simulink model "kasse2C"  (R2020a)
settings: Solver=ode45  StartTime=0.0  StopTime=100  FixedStep=0.001  MaxStep=2  RelTol=1e-3  EnableMultiTasking=on
libraries: simulink x2

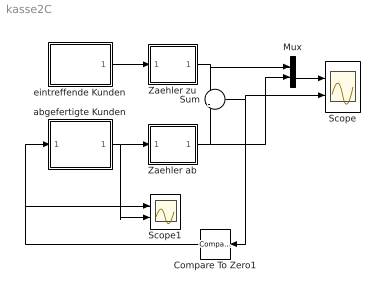
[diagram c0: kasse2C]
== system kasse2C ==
  Compare To Zero1 : simulink/Logic and Bit Operations/Compare To Zero  relop=<=  OutDataTypeStr=uint8
  Mux : Mux  Inputs=2
  Scope : Scope  NumInputPorts=2
  Scope1 : Scope  NumInputPorts=2
  Sum : Sum  Inputs=+|-
  Zaehler ab : Subsystem  mask(Vorwaertszaehler){z0=0}
      mask prompts: z0 "Anfangswert"
      mask help: Einfacher Vorwaertszaehler, getriggert durch Signalabfall
  Zaehler zu : Subsystem  mask(Vorwaertszaehler){z0=0}
      mask prompts: z0 "Anfangswert"
      mask help: Einfacher Vorwaertszaehler, getriggert durch Signalabfall
  abgefertigte Kunden : Subsystem  mask{tAb=1}
      mask prompts: tAb "Abfertigungszeit [s]"
  eintreffende Kunden : Subsystem  mask(Poisson-Impulse){lambda=0.8}
      mask help: Erzeugt Impulse, deren zeitlicher Abstand exponentialverteilt ist mit Rate lambda. Summiert man die Anzahl der Impulse, erhaelt man einen Poisson-Prozess.
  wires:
  Zaehler zu/1(Out) -> Sum/1, Mux/1
  eintreffende Kunden/1(Out1) -> Zaehler zu/1(In)
  abgefertigte Kunden/1(Out) -> Scope1/2, Zaehler ab/1(In)
  Zaehler ab/1(Out) -> Sum/2, Mux/2
  Sum/1 -> Compare To Zero1/1, Scope/2
  Compare To Zero1/1 -> abgefertigte Kunden/1(In1), Scope1/1
  Mux/1 -> Scope/1

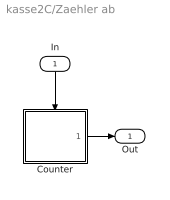
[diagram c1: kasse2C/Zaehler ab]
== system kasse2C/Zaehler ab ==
  In : Inport
  Counter : Subsystem
  Out : Outport
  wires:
  Counter/1(Out) -> Out/1
  In/1 -> Counter/Trigger

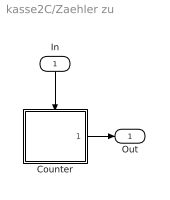
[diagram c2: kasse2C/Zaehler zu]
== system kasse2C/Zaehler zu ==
  In : Inport
  Counter : Subsystem
  Out : Outport
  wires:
  In/1 -> Counter/Trigger
  Counter/1(Out) -> Out/1

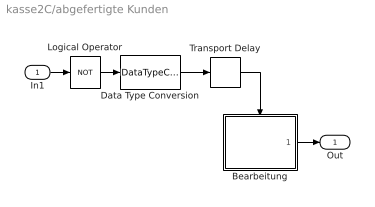
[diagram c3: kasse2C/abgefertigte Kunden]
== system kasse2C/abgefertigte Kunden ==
  In1 : Inport
  Bearbeitung : Subsystem
  Data Type Conversion : DataTypeConversion  OutDataTypeStr=double
  Logical Operator : Logic  Operator=NOT  AllPortsSameDT=off  OutDataTypeStr=boolean
  Transport Delay : TransportDelay  DelayTime=0.2*tAb
  Out : Outport
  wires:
  In1/1 -> Logical Operator/1
  Bearbeitung/1(Out1) -> Out/1
  Logical Operator/1 -> Data Type Conversion/1
  Data Type Conversion/1 -> Transport Delay/1
  Transport Delay/1 -> Bearbeitung/Enable

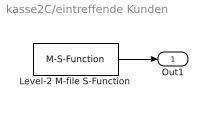
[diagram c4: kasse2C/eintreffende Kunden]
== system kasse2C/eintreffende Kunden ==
  Level-2 M-file S-Function : M-S-Function  FunctionName=sfun_poisson  Parameters=lambda
  Out1 : Outport
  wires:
  Level-2 M-file S-Function/1 -> Out1/1

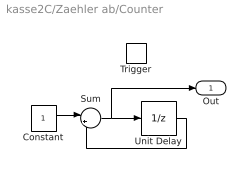
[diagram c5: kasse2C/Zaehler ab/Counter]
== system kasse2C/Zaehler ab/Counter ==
  Trigger : TriggerPort  TriggerType=falling  VariantControl=Variant
  Constant : Constant
  Sum : Sum  Inputs=|++
  Unit Delay : UnitDelay  InitialCondition=z0  SampleTime=-1  HasFrameUpgradeWarning=on
  Out : Outport  InitialOutput=z0
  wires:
  Constant/1 -> Sum/1
  Sum/1 -> Unit Delay/1, Out/1
  Unit Delay/1 -> Sum/2

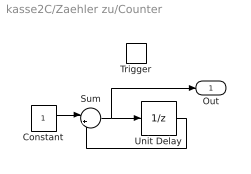
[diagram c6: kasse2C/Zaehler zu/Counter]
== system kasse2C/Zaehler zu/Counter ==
  Trigger : TriggerPort  TriggerType=falling  VariantControl=Variant
  Constant : Constant
  Sum : Sum  Inputs=|++
  Unit Delay : UnitDelay  InitialCondition=z0  SampleTime=-1  HasFrameUpgradeWarning=on
  Out : Outport  InitialOutput=z0
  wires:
  Unit Delay/1 -> Sum/2
  Sum/1 -> Out/1, Unit Delay/1
  Constant/1 -> Sum/1

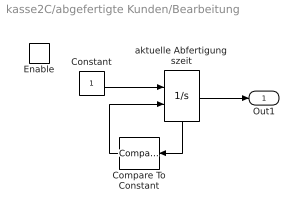
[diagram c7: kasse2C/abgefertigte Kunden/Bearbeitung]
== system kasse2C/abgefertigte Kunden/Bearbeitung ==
  Enable : EnablePort  StatesWhenEnabling=reset
  Compare To Constant : simulink/Logic and Bit Operations/Compare To Constant  relop=>=  const=tAb  OutDataTypeStr=boolean
  Constant : Constant
  aktuelle Abfertigungszeit : Integrator  ExternalReset=rising  ShowStatePort=on
  Out1 : Outport  OutputWhenDisabled=reset  InitialOutput=0
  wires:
  Compare To Constant/1 -> aktuelle Abfertigungszeit/2
  aktuelle Abfertigungszeit/1 -> Out1/1
  Constant/1 -> aktuelle Abfertigungszeit/1
  aktuelle Abfertigungszeit/State -> Compare To Constant/1
